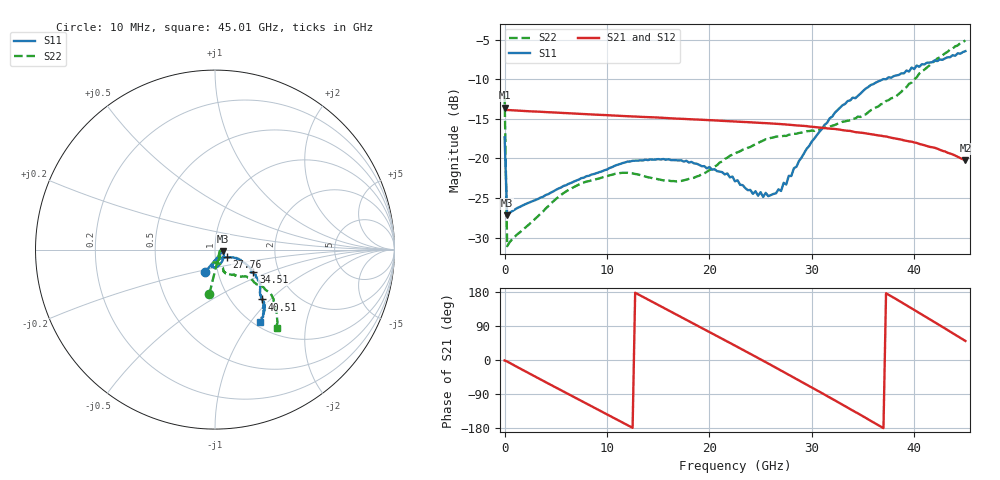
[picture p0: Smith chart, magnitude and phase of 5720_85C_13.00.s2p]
! Device:  ADRF5720
! Description: 0.5dB LSB GaAs MMIC 6-bit Digital Attenuator
! Frequency:  0.000009 -  40 GHz
! Ports:
!	RF1	= Port 1
!	RF2	= Port 2
! Vdd:  3.3 Volt
! Vss:  -3.3 Volt
! Control:  0/3.3 Volt
! State:  13.00 dB attenuation
! Data:  The device was measured using G-S-G Probes on a matrix board.
!  Data was collected using an calibrated 4 port network analyzer.
!  The reference plane for this measurement is at the launchers.
! Note:  Analog Devices supplies this data as a sample of measured data
!  for this product.  Your particular data for this product may vary.
!  Data was taken at 85 degrees C.
!  Analog Devices reserves the right to change this data at anytime.
# GHZ S DB R 45.0
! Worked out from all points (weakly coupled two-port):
!   181 points, 10 MHz to 45.01 GHz, reference 45 ohm
!   highest |S21| = -13.57 dB at 10 MHz (marker M1); lowest = -20.2 dB at 45.01 GHz (marker M2)
!   lowest |S11| = -27.2 dB at 260 MHz (marker M3), VSWR 1.09, Z = 49 - j0.845 ohm
!   |S11| at or under -10 dB: start of sweep to 36.95 GHz
!   |S22| runs from -31.1 to -5.1 dB; largest |S21 - S12| = 0.00094
!   S11 on the Smith chart (normalised r, x): 10 MHz: 0.87, -0.22; 27.76 GHz: 1.13, -0.10; 34.51 GHz: 1.48, -0.40; 40.51 GHz: 1.37, -0.89; 45.01 GHz: 1.07, -1.12
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0.01  -17.32 -113.8  -13.57 -1.3  -13.56 -1.3  -12.07 -97.2
0.26  -27.20 -11.4  -13.87 -4.0  -13.86 -4.0  -31.09 -17.6
4.26  -24.52 -35.3  -14.15 -61.9  -14.13 -61.8  -26.04 -57.4
7.76  -22.42 -58.2  -14.38 -111.6  -14.37 -111.6  -23.04 -81.0
11.76  -20.51 -79.5  -14.64 -168.3  -14.63 -168.2  -21.81 -96.1
15.26  -20.13 -93.2  -14.85 141.8  -14.83 142.0  -22.69 -96.1
19.01  -20.81 -99.9  -15.09 88.3  -15.07 88.5  -22.19 -76.9
22.76  -22.76 -93.3  -15.35 34.3  -15.33 34.5  -19.22 -67.5
25.26  -24.87 -73.7  -15.52 -2.0  -15.50 -1.8  -17.74 -67.7
27.01  -24.11 -44.7  -15.65 -27.8  -15.64 -27.5  -17.21 -66.4
27.51  -23.30 -37.9  -15.71 -35.2  -15.70 -34.9  -17.15 -66.1
27.76  -22.20 -33.7  -15.73 -38.9  -15.72 -38.6  -17.00 -66.7
28.01  -22.22 -33.3  -15.76 -42.7  -15.75 -42.4  -17.01 -66.1
28.26  -21.23 -29.2  -15.79 -46.3  -15.77 -46.0  -16.88 -66.4
30.26  -17.48 -23.3  -16.02 -76.2  -16.00 -75.9  -16.52 -63.3
32.51  -13.90 -26.0  -16.31 -110.3  -16.30 -110.1  -15.62 -57.2
34.51  -12.09 -30.4  -16.70 -140.8  -16.69 -140.5  -14.71 -52.0
35.76  -10.72 -34.8  -16.92 -160.4  -16.90 -160.1  -13.91 -47.9
37.76  -9.79 -39.4  -17.38 168.2  -17.36 168.5  -12.39 -40.3
40.51  -8.41 -47.0  -18.16 123.9  -18.13 124.3  -9.26 -37.8
42.26  -7.69 -49.4  -18.76 95.6  -18.74 95.9  -7.37 -40.3
45.01  -6.43 -58.1  -20.25 50.3  -20.22 50.6  -5.08 -52.0
